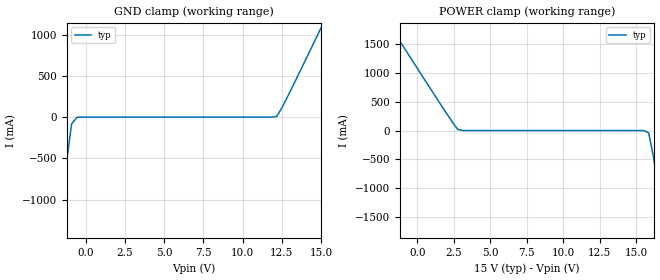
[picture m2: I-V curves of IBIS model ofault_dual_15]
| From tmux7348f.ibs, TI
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| ofault_dual_15
[Model]   ofault_dual_15
Model_type   Input
Vinl = 0.8
Vinh = 1.3
|   typ   min   max
C_comp   2.533030e-12   NA   NA
[Voltage Range]   15   NA   NA
[Temperature Range]   27   NA   NA
[Power Clamp Reference]   15   NA   NA
[GND Clamp Reference]   0   NA   NA
[GND Clamp]
|   Voltage   I(typ)   I(min)   I(max)
-20V      -251.7A    NA         NA
-1.97V    -1.757A    NA         NA
-1.616V   -1.163A    NA         NA
-1.263V   -583.9mA   NA         NA
-909.1mV  -80.83mA   NA         NA
-555.6mV  -2.017mA   NA         NA
11.82V    32.41nA    NA         NA
12.17V    8.054mA    NA         NA
12.53V    120.6mA    NA         NA
12.88V    253.9mA    NA         NA
15V       1.085A     NA         NA
[POWER Clamp]
|   Voltage   I(typ)   I(min)   I(max)
-5V       3.067A     NA         NA
-1.818V   1.804A     NA         NA
1.717V    410.1mA    NA         NA
2.778V    19.05mA    NA         NA
3.131V    161.6nA    NA         NA
15.51V    -880.2uA   NA         NA
15.86V    -42.96mA   NA         NA
16.21V    -503.8mA   NA         NA
16.92V    -1.671A    NA         NA
17.27V    -2.271A    NA         NA
30V       -179.9A    NA         NA
